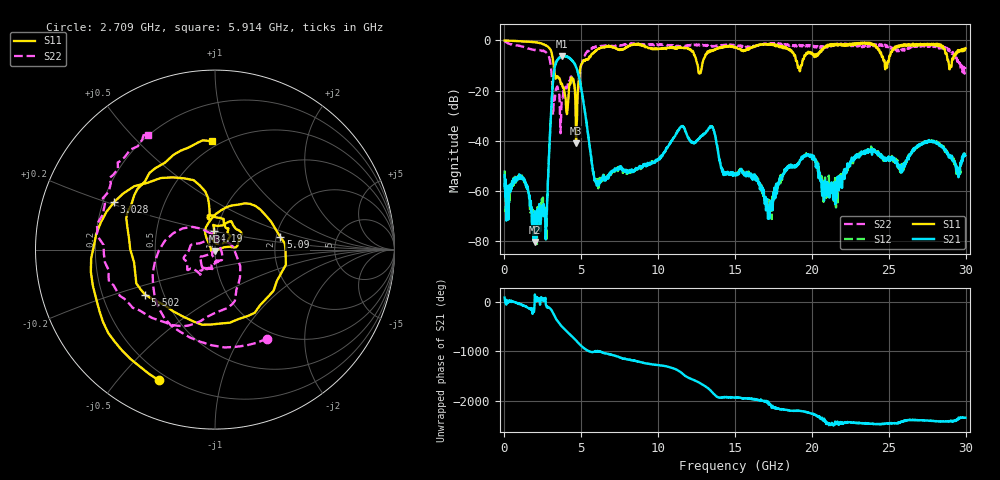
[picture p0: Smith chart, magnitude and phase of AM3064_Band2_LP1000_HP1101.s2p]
# Hz S DB R 50.0
!freq dBS11 angS11 dBS21 angS21 dBS12 angS12 dBS22 angS22
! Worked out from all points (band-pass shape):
!   1600 points, 10 MHz to 29.98 GHz, reference 50 ohm
!   highest |S21| = -6.24 dB at 3.759 GHz (marker M1); lowest = -80.3 dB at 1.959 GHz (marker M2)
!   |S21| within 3 dB of the highest: 3.332 GHz to 4.552 GHz (1.22 GHz wide, 31 % of centre)
!   lowest |S11| = -41.0 dB at 4.658 GHz (marker M3), VSWR 1.02, Z = 50.1 - j0.885 ohm
!   |S11| at or under -10 dB: 3.202 GHz to 4.97 GHz (1.768 GHz wide, 43.3 % of centre); 12.57 GHz to 12.86 GHz (288 MHz wide, 2.27 % of centre); 19.06 GHz to 19.3 GHz (231.3 MHz wide, 1.21 % of centre)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
!   |S22| runs from -37.0 to -0.3 dB; largest |S21 - S12| = 0.017
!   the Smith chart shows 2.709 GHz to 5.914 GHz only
!   S11 on the Smith chart (normalised r, x): 2.709 GHz: 0.17, -0.64; 3.028 GHz: 0.24, +0.21; 4.19 GHz: 0.97, +0.20; 5.09 GHz: 2.11, +0.34; 5.502 GHz: 0.39, -0.25; 5.914 GHz: 0.46, +0.87
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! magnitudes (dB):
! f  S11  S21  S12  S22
! 10 MHz  0.0  -53.6  -51.8  -0.3
! 1.228 GHz  -0.5  -55.0  -55.4  -2.6
! 1.959 GHz  -0.8  -80.3  -75.3  -3.9
! 2.709 GHz  -2.0  -75.7  -70.0  -4.8
! 3.028 GHz  -4.1  -29.2  -29.2  -11.0
! 3.29 GHz  -14.7  -10.1  -10.2  -22.6
! 3.759 GHz  -17.7  -6.2  -6.4  -23.0
! 4.19 GHz  -19.6  -6.8  -7.0  -15.8
! 4.658 GHz  -41.0  -10.7  -10.5  -20.8
! 5.015 GHz  -9.4  -19.8  -19.7  -9.6
! 5.09 GHz  -8.6  -22.6  -22.6  -7.8
! 5.502 GHz  -6.7  -40.4  -40.2  -4.1
! 5.914 GHz  -4.4  -56.2  -55.5  -2.6
! 10 GHz  -3.4  -47.2  -47.6  -1.8
! 13.43 GHz  -4.4  -34.2  -34.1  -2.4
! 14.18 GHz  -2.6  -51.2  -52.2  -2.0
! 15 GHz  -2.6  -53.5  -53.6  -1.9
! 17.25 GHz  -1.5  -68.9  -63.8  -1.2
! 19.99 GHz  -5.0  -45.6  -46.2  -2.0
! 20.91 GHz  -2.3  -59.8  -56.4  -2.4
! 25 GHz  -8.2  -46.2  -48.0  -2.2
! 29.98 GHz  -3.2  -45.8  -45.4  -10.6
